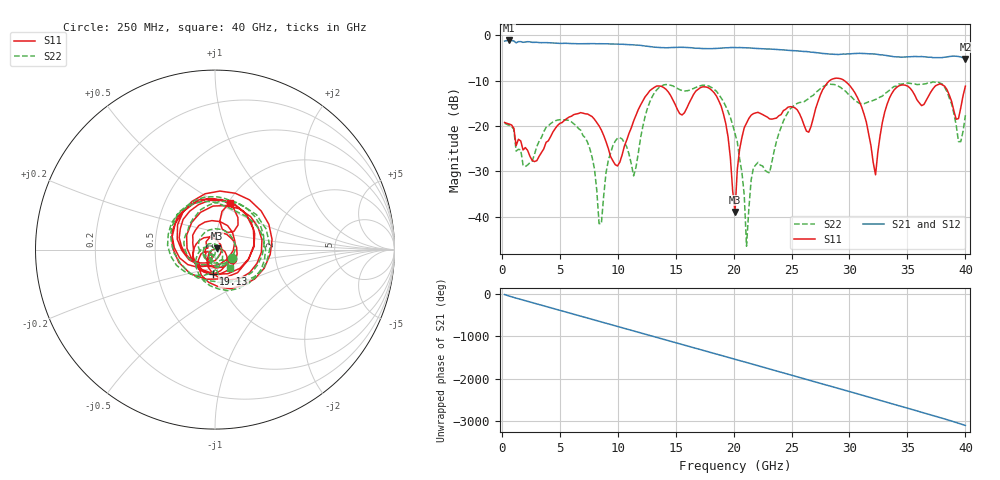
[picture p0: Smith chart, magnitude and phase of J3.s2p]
!Agilent Technologies,E8364B,MY43040528,A.07.50.67
!Agilent E8364B: A.07.50.67
!Date: Thursday, May 22, 2025 21:04:16
!Correction: S11(Full 2 Port(1,2))
!S21(Full 2 Port(1,2))
!S12(Full 2 Port(1,2))
!S22(Full 2 Port(1,2))
!S2P File: Measurements: S11, S21, S12, S22:
# Hz S  dB  R 50
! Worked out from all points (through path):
!   201 points, 250 MHz to 40 GHz, reference 50 ohm
!   highest |S21| = -1.13 dB at 647.5 MHz (marker M1); lowest = -5.2 dB at 40 GHz (marker M2)
!   group delay of S21, straight-line fit = 214 ps
!   lowest |S11| = -39.0 dB at 20.12 GHz (marker M3), VSWR 1.02, Z = 50.9 + j0.694 ohm
!   |S11| at or under -10 dB: start of sweep to 28.28 GHz; 29.56 GHz to end of sweep
!   |S22| runs from -46.5 to -10.3 dB; largest |S21 - S12| = 0.0057
!   S11 on the Smith chart (normalised r, x): 250 MHz: 1.20, -0.13; 19.13 GHz: 0.94, -0.26; 40 GHz: 1.02, +0.58
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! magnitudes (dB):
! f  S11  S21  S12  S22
! 250 MHz  -19.2  -1.3  -1.3  -19.4
! 647.5 MHz  -19.6  -1.1  -1.2  -19.9
! 2.834 GHz  -27.8  -1.5  -1.5  -26.2
! 4.622 GHz  -20.5  -1.7  -1.7  -18.9
! 7.008 GHz  -17.2  -1.9  -1.9  -22.1
! 8.598 GHz  -20.9  -1.9  -1.9  -41.6
! 9.591 GHz  -27.7  -1.9  -1.9  -24.3
! 11.38 GHz  -18.9  -2.1  -2.1  -31.0
! 13.57 GHz  -11.2  -2.7  -2.7  -11.5
! 19.13 GHz  -17.4  -2.8  -2.8  -14.6
! 20.12 GHz  -39.0  -2.7  -2.7  -21.7
! 20.92 GHz  -20.4  -2.7  -2.8  -35.1
! 21.12 GHz  -19.4  -2.8  -2.8  -46.5
! 21.71 GHz  -17.3  -2.9  -2.9  -29.2
! 23.11 GHz  -18.4  -3.0  -3.1  -30.3
! 26.88 GHz  -18.2  -3.7  -3.8  -13.2
! 29.86 GHz  -10.7  -4.1  -4.1  -12.9
! 32.25 GHz  -30.8  -4.1  -4.2  -14.1
! 33.44 GHz  -13.9  -4.6  -4.6  -12.1
! 38.01 GHz  -10.9  -4.9  -4.9  -10.8
! 39.2 GHz  -18.5  -4.6  -4.6  -19.8
! 40 GHz  -11.2  -5.2  -5.2  -17.6
